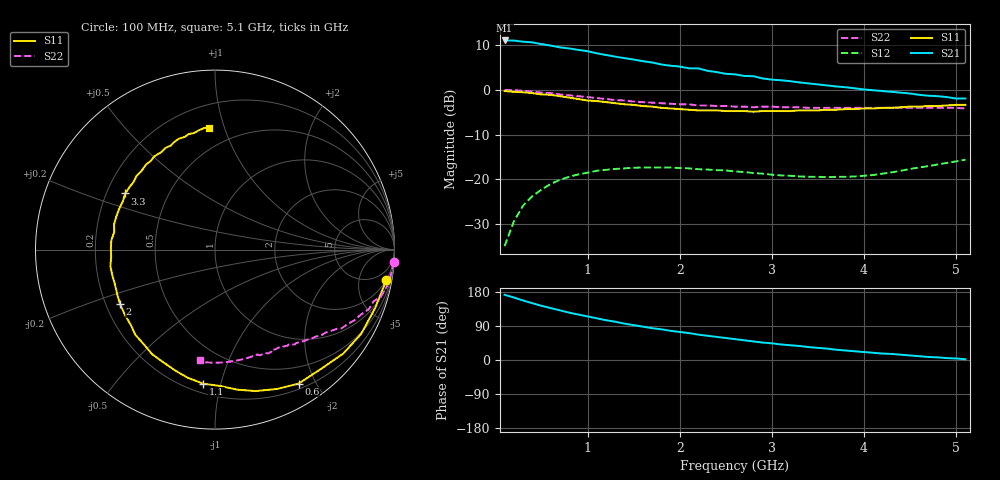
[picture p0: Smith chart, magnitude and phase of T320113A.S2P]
!AT-32011
!S PARAMETERS at Vce=2.7 V  Ic=1mA.  LAST UPDATED 01-05-95
# ghz s ma r 50
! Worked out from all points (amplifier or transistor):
!   51 points, 100 MHz to 5.1 GHz, reference 50 ohm
!   highest |S21| = 11.0 dB at 100 MHz (marker M1)
!   |S21| within 3 dB of that: start of sweep to 1.136 GHz
!   unconditionally stable (mu >= 1): 2.754 GHz to end of sweep
!   at 900 MHz: K = 0.29, MSG = 13.9 dB, |S12| = -18.9 dB
!   at 2.6 GHz: K = 0.92, MSG = 10.8 dB, |S12| = -18.2 dB
!   at 5.1 GHz: K = 1.04, MAG = 5.7 dB, |S12| = -15.6 dB
!   S11 on the Smith chart (normalised r, x): 100 MHz: 2, -11; 600 MHz: 0.27, -1.77; 1.1 GHz: 0.26, -0.88; 2 GHz: 0.26, -0.25; 3.3 GHz: 0.28, +0.27; 5.1 GHz: 0.35, +0.89
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0.1  0.97 -10.0  3.56 172.0  0.018 84.0  1 -4.0
0.2  0.95 -20.0  3.55 165.0  0.034 78.0  0.99 -8.0
0.3  0.94 -30.0  3.45 157.0  0.051 72.0  0.98 -12.0
0.4  0.92 -39.0  3.39 150.0  0.065 66.0  0.96 -16.0
0.5  0.89 -48.0  3.24 143.0  0.077 61.0  0.93 -18.0
0.6  0.88 -58.0  3.12 137.0  0.089 56.0  0.92 -21.0
0.8  0.82 -74.0  2.9 125.0  0.107 47.0  0.87 -27.0
1  0.76 -88.0  2.7 115.0  0.119 40.0  0.83 -32.0
1.1  0.75 -95.0  2.56 110.0  0.125 37.0  0.81 -33.0
1.4  0.69 -115.0  2.26 96.0  0.133 28.0  0.76 -39.0
1.7  0.65 -133.0  2.02 84.0  0.136 21.0  0.72 -44.0
1.8  0.63 -138.0  1.92 81.0  0.136 20.0  0.71 -46.0
2  0.61 -150.0  1.82 74.0  0.134 17.0  0.69 -49.0
2.1  0.6 -155.0  1.74 71.0  0.133 15.0  0.69 -50.0
2.2  0.59 -161.0  1.74 67.0  0.13 14.0  0.67 -52.0
2.3  0.59 -166.0  1.63 64.0  0.129 13.0  0.67 -53.0
2.6  0.58 179.0  1.49 55.0  0.123 12.0  0.65 -57.0
2.9  0.58 166.0  1.34 46.0  0.116 12.0  0.65 -61.0
3.3  0.59 148.0  1.21 37.0  0.108 16.0  0.64 -67.0
3.5  0.59 140.0  1.15 32.0  0.107 20.0  0.63 -70.0
4.3  0.63 113.0  0.95 16.0  0.12 37.0  0.63 -82.0
5.1  0.68 93.0  0.8 2.0  0.166 42.0  0.62 -98.0
